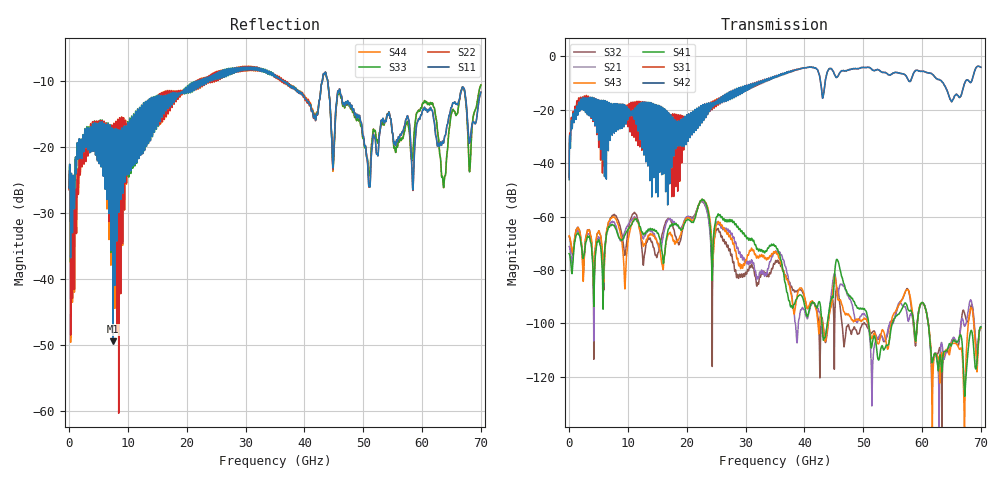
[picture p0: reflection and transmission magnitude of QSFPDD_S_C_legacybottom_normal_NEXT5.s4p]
! AWR Design Environment (8415) Thu Dec 20 14:58:06 2018
! Document = 'CHANNEL TEST'
! nPorts: 4, nXvals: 7001
# HZ S DB R 50
!Freq DBS11 AngS11 DBS12 AngS12 DBS13 AngS13 DBS14 AngS14
!	DBS21 AngS21 DBS22 AngS22 DBS23 AngS23 DBS24 AngS24
!	DBS31 AngS31 DBS32 AngS32 DBS33 AngS33 DBS34 AngS34
!	DBS41 AngS41 DBS42 AngS42 DBS43 AngS43 DBS44 AngS44
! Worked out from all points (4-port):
!   7000 points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, 10 MHz to 70 GHz, reference 50 ohm
!   strongest paths, dB at 10 MHz, 17.51 GHz, 35.01 GHz, 52.51 GHz, 70 GHz:
!     S42: -46.2, -26.2, -7.4, -5.0, -4.0
!     S31: -45.3, -28.7, -7.5, -5.0, -4.0
!     S41: -73.9, -62.7, -71.0, -113.3, -101.3
!     S43: -67.2, -67.0, -73.4, -107.6, -101.7
!     S21: -71.2, -61.2, -73.4, -105.4, -101.2
!     S32: -67.6, -62.4, -77.3, -105.9, -101.8
!   lowest |S11| = -49.4 dB at 7.45 GHz (marker M1), VSWR 1.01, Z = 50.3 + j0.0931 ohm
!   |S11| at or under -10 dB: start of sweep to 22.1 GHz; 36.25 GHz to 43.06 GHz (6.813 GHz wide, 17.2 % of centre); 43.96 GHz to end of sweep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
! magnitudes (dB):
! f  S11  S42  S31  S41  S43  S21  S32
! 10 MHz  -26.2  -46.2  -45.3  -73.9  -67.2  -71.2  -67.6
! 1.64 GHz  -19.9  -17.2  -15.5  -66.7  -64.8  -65.7  -64.6
! 7.45 GHz  -49.4  -18.2  -18.5  -63.1  -60.2  -61.9  -59.5
! 9.49 GHz  -24.4  -18.2  -19.0  -66.9  -87.1  -65.6  -74.5
! 22.66 GHz  -10.7  -19.6  -21.8  -53.5  -53.6  -54.2  -54.3
! 28.46 GHz  -8.2  -12.8  -13.0  -63.6  -75.1  -71.3  -82.7
! 70 GHz  -11.8  -4.0  -4.0  -101.3  -101.7  -101.2  -101.8
